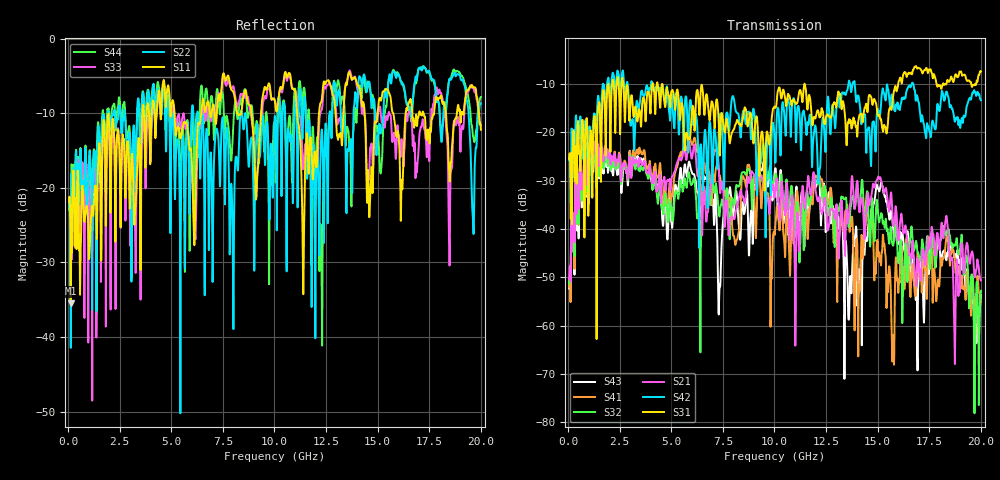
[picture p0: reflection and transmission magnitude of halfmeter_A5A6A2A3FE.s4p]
! FILE: D:\iPass\iPassCable1005\iPassCable\SOLT_cal\halfmeter_A5A6A2A3FE.s4p
# MHz S MA R 50.00
! FREQ  S11  S12  S13  S14
!  S21  S22  S23  S24
!  S31  S32  S33  S34
!  S41  S42  S43  S44
!  MAG  ANG  MAG  ANG  MAG  ANG  MAG  ANG
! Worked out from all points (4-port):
!   1996 points, 50 MHz to 20 GHz, reference 50 ohm
!   strongest paths, dB at 50 MHz, 5.04 GHz, 10.03 GHz, 15.02 GHz, 20 GHz:
!     S31: -25.5, -11.3, -14.9, -16.5, -7.4
!     S42: -25.8, -13.5, -25.5, -15.4, -13.3
!     S21: -50.3, -29.1, -33.0, -29.1, -50.6
!     S32: -51.3, -38.1, -29.2, -36.9, -52.8
!     S41: -51.9, -33.0, -40.1, -44.8, -55.1
!     S43: -52.3, -39.8, -27.6, -31.7, -53.6
!   lowest |S11| = -35.5 dB at 130 MHz (marker M1), VSWR 1.03, Z = 51.1 - j1.33 ohm
!   |S11| at or under -10 dB: start of sweep to 3.596 GHz; 5.151 GHz to 6.452 GHz (1.301 GHz wide, 22.4 % of centre); 11.09 GHz to 12.16 GHz (1.066 GHz wide, 9.17 % of centre)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
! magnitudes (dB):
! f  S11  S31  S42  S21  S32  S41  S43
! 50 MHz  -21.9  -25.5  -25.8  -50.3  -51.3  -51.9  -52.3
! 130 MHz  -35.5  -37.9  -34.6  -50.9  -50.9  -51.6  -51.9
! 5.9 GHz  -15.0  -21.3  -13.7  -22.7  -29.6  -21.0  -26.5
! 7.33 GHz  -7.9  -22.4  -17.6  -30.2  -37.4  -29.0  -52.4
! 9.48 GHz  -7.0  -24.7  -23.4  -30.3  -28.9  -29.3  -26.0
! 12.25 GHz  -8.6  -16.2  -23.4  -36.1  -31.5  -29.6  -39.3
! 20 GHz  -12.2  -7.4  -13.3  -50.6  -52.8  -55.1  -53.6
